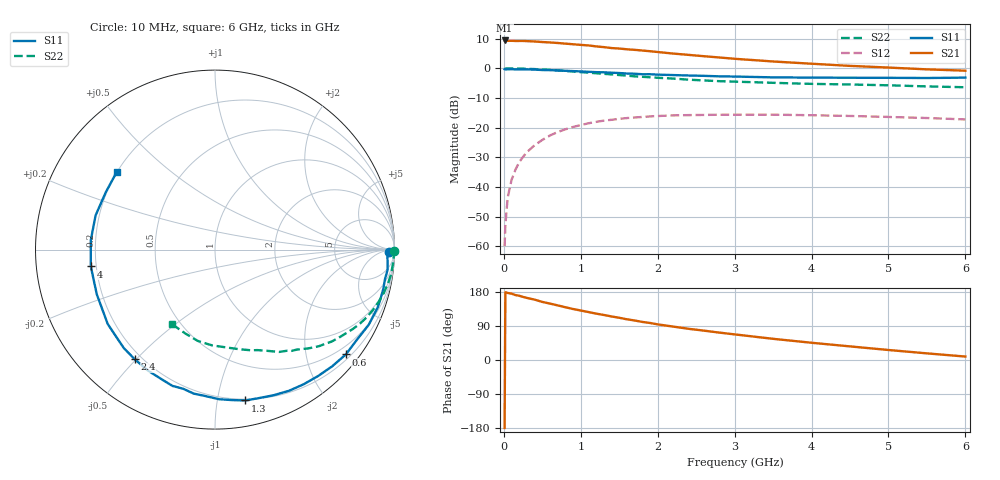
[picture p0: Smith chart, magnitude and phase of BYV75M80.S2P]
! SIEMENS Small Signal Semiconductors
! BFY420
! Si NPN RF SIEGET Grounded Emitter Transistor in MICRO-X
! VCE = 0.75 V  IC = 0.8 mA
! Common Emitter S-Parameters:  October  1996
# GHz  S  MA  R  50
!  f  S11  S21  S12  S22
! GHz  MAG  ANG  MAG  ANG  MAG  ANG  MAG  ANG
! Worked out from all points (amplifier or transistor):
!   36 points, 10 MHz to 6 GHz, reference 50 ohm
!   highest |S21| = 9.4 dB at 10 MHz (marker M1)
!   |S21| within 3 dB of that: start of sweep to 1.611 GHz
!   unconditionally stable (mu >= 1): 4.647 GHz to end of sweep
!   at 250 MHz: K = 0.04, MSG = 19.6 dB, |S12| = -29.9 dB
!   at 1.4 GHz: K = 0.23, MSG = 12.1 dB, |S12| = -17.4 dB
!   at 6 GHz: K = 1.35, MAG = 4.7 dB, |S12| = -17.2 dB
!   S11 on the Smith chart (normalised r, x): 10 MHz: 53, -23; 600 MHz: 0.31, -2.82; 1.3 GHz: 0.19, -1.20; 2.4 GHz: 0.17, -0.50; 4 GHz: 0.18, -0.07; 6 GHz: 0.20, +0.33
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0.01  0.9686 -0.8  2.955 -179.4  0.001 93.7  0.9978 -0.4
0.02  0.9603 -1.3  2.936 178.8  0.0023 86.2  0.991 -0.6
0.05  0.9632 -3.6  2.91 176.9  0.0066 88.1  0.997 -1.8
0.1  0.968 -6.7  2.916 175.1  0.0131 86.6  0.9953 -3.6
0.15  0.9613 -9.9  2.895 171.4  0.0194 83.2  0.9932 -5.5
0.3  0.9621 -19.5  2.878 163.8  0.0386 77.4  0.9829 -10.9
0.4  0.9533 -26.1  2.841 159.4  0.0505 73.2  0.9715 -14.3
0.5  0.9365 -32.5  2.78 153.2  0.062 69.2  0.957 -17.8
0.6  0.9341 -38.7  2.734 148.9  0.0737 64.9  0.9415 -21.1
0.9  0.8983 -56.6  2.549 134.5  0.1027 53.4  0.8851 -30.1
1.1  0.8744 -68.2  2.436 126.5  0.1184 46.6  0.8458 -35.6
1.3  0.8574 -78.6  2.279 118.8  0.1312 40.2  0.8082 -40.5
1.6  0.8178 -93.7  2.097 107.4  0.1449 31.8  0.7529 -47.1
1.8  0.7952 -102.9  1.999 100.5  0.1513 26.9  0.7199 -50.7
2.2  0.7706 -119.0  1.776 88.2  0.1609 17.9  0.6724 -58.0
2.4  0.7572 -126.2  1.688 82.4  0.1626 14.4  0.6441 -61.4
2.8  0.733 -139.2  1.526 72.3  0.1649 7.7  0.6073 -67.2
3.5  0.7042 -159.3  1.306 55.9  0.1654 -1.3  0.5699 -76.7
4  0.6982 -172.3  1.197 45.5  0.1618 -6.7  0.5471 -84.0
4.5  0.694 175.7  1.101 35.9  0.1573 -11.6  0.5341 -91.7
5.5  0.6872 152.3  0.962 17.5  0.1452 -17.6  0.4958 -109.5
6  0.6975 141.8  0.913 9.1  0.1375 -18.5  0.4797 -119.7
